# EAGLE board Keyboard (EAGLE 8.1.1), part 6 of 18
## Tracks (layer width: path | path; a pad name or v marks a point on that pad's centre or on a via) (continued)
S$5418 (continued)
  Bottom 0: 86.17,47.48 86.18,47.38
S$5419
  Bottom 0: 86.18,47.38 86.2,47.3
S$5420
  Bottom 0: 86.2,47.3 86.24,47.22
S$5421
  Bottom 0: 86.24,47.22 86.28,47.14
S$5422
  Bottom 0: 86.28,47.14 86.34,47.07
S$5423
  Bottom 0: 86.34,47.07 90.51,42.91
S$5424
  Bottom 0: 90.51,42.91 89.52,41.92
S$5425
  Bottom 0: 89.52,41.92 89.54,42.08
S$5426
  Bottom 0: 89.54,42.08 89.5,42.38
S$5427
  Bottom 0: 89.5,42.38 89.36,42.65
S$5428
  Bottom 0: 89.36,42.65 89.16,42.87
S$5429
  Bottom 0: 89.16,42.87 88.9,43.02
S$5430
  Bottom 0: 88.9,43.02 88.6,43.09
S$5431
  Bottom 0: 88.6,43.09 88.3,43.07
S$5432
  Bottom 0: 88.3,43.07 88.02,42.96
S$5433
  Bottom 0: 88.02,42.96 87.78,42.77
S$5434
  Bottom 0: 87.78,42.77 87.61,42.52
S$5435
  Bottom 0: 87.61,42.52 87.52,42.23
S$5436
  Bottom 0: 87.52,42.23 87.52,41.92
S$5437
  Bottom 0: 87.52,41.92 87.61,41.64
S$5438
  Bottom 0: 87.61,41.64 87.78,41.39
S$5439
  Bottom 0: 87.78,41.39 88.02,41.2
S$5440
  Bottom 0: 88.02,41.2 88.3,41.09
S$5441
  Bottom 0: 88.3,41.09 88.6,41.07
S$5442
  Bottom 0: 88.6,41.07 88.9,41.13
S$5443
  Bottom 0: 88.9,41.13 89.16,41.28
S$5444
  Bottom 0: 89.16,41.28 89.22,41.35
S$5445
  Bottom 0: 89.22,41.35 89.22,32.67
S$5446
  Bottom 0: 89.22,32.67 89.04,32.55
S$5447
  Bottom 0: 89.04,32.55 88.83,32.31
S$5448
  Bottom 0: 88.83,32.31 88.69,32.01
S$5449
  Bottom 0: 88.69,32.01 88.64,31.69
S$5450
  Bottom 0: 88.64,31.69 88.69,31.37
S$5451
  Bottom 0: 88.69,31.37 88.83,31.07
S$5452
  Bottom 0: 88.83,31.07 89.04,30.82
S$5453
  Bottom 0: 89.04,30.82 89.17,30.74
S$5454
  Bottom 0: 89.17,30.74 88.38,30.74
S$5455
  Bottom 0: 88.38,30.74 88.39,30.8
S$5456
  Bottom 0: 88.39,30.8 88.39,32.58
S$5457
  Bottom 0: 88.39,32.58 88.38,32.65
S$5458
  Bottom 0: 88.38,32.65 88.34,32.72
S$5459
  Bottom 0: 88.34,32.72 88.28,32.78
S$5460
  Bottom 0: 88.28,32.78 88.21,32.82
S$5461
  Bottom 0: 88.21,32.82 88.14,32.83
S$5462
  Bottom 0: 88.14,32.83 87.69,32.83
S$5463
  Bottom 0: 87.69,32.83 87.69,32.96
S$5464
  Bottom 0: 87.69,32.96 87.63,33.18
S$5465
  Bottom 0: 87.63,33.18 87.47,33.34
S$5466
  Bottom 0: 87.47,33.34 87.25,33.4
S$5467
  Bottom 0: 87.25,33.4 86.89,33.4
S$5468
  Bottom 0: 86.89,33.4 85.8,34.48
S$5469
  Bottom 0: 85.8,34.48 85.86,34.62
S$5470
  Bottom 0: 85.86,34.62 85.91,34.94
S$5471
  Bottom 0: 85.91,34.94 85.86,35.26
S$5472
  Bottom 0: 85.86,35.26 85.73,35.56
S$5473
  Bottom 0: 85.73,35.56 85.53,35.81
S$5474
  Bottom 0: 85.53,35.81 85.27,36
S$5475
  Bottom 0: 85.27,36 84.96,36.11
S$5476
  Bottom 0: 84.96,36.11 84.64,36.13
S$5477
  Bottom 0: 84.64,36.13 84.31,36.06
S$5478
  Bottom 0: 84.31,36.06 84.02,35.91
S$5479
  Bottom 0: 84.02,35.91 83.79,35.69
S$5480
  Bottom 0: 83.79,35.69 83.62,35.41
S$5481
  Bottom 0: 83.62,35.41 83.53,35.1
S$5482
  Bottom 0: 83.53,35.1 83.53,34.77
S$5483
  Bottom 0: 83.53,34.77 83.62,34.46
S$5484
  Bottom 0: 83.62,34.46 83.79,34.19
S$5485
  Bottom 0: 83.79,34.19 84.02,33.96
S$5486
  Bottom 0: 84.02,33.96 84.31,33.81
S$5487
  Bottom 0: 84.31,33.81 84.64,33.75
S$5488
  Bottom 0: 84.64,33.75 84.96,33.77
S$5489
  Bottom 0: 84.96,33.77 85.18,33.85
S$5490
  Bottom 0: 85.18,33.85 86.24,32.79
S$5491
  Bottom 0: 86.24,32.79 86.21,32.78
S$5492
  Bottom 0: 86.21,32.78 86.15,32.72
S$5493
  Bottom 0: 86.15,32.72 86.11,32.65
S$5494
  Bottom 0: 86.11,32.65 86.1,32.58
S$5495
  Bottom 0: 86.1,32.58 86.1,30.8
S$5496
  Bottom 0: 86.1,30.8 86.11,30.74
S$5497
  Bottom 0: 86.11,30.74 80,30.74
S$5498
  Bottom 0: 80,30.74 79.97,30.95
S$5499
  Bottom 0: 79.97,30.95 79.83,31.22
S$5500
  Bottom 0: 79.83,31.22 79.63,31.44
S$5501
  Bottom 0: 79.63,31.44 79.37,31.59
S$5502
  Bottom 0: 79.37,31.59 79.07,31.66
S$5503
  Bottom 0: 79.07,31.66 78.77,31.64
S$5504
  Bottom 0: 78.77,31.64 78.49,31.53
S$5505
  Bottom 0: 78.49,31.53 78.25,31.34
S$5506
  Bottom 0: 78.25,31.34 78.08,31.09
S$5507
  Bottom 0: 78.08,31.09 77.99,30.8
S$5508
  Bottom 0: 77.99,30.8 77.99,30.5
S$5509
  Bottom 0: 77.99,30.5 78.08,30.21
S$5510
  Bottom 0: 78.08,30.21 78.25,29.96
S$5511
  Bottom 0: 78.25,29.96 78.49,29.77
S$5512
  Bottom 0: 78.49,29.77 78.77,29.66
S$5513
  Bottom 0: 78.77,29.66 79.07,29.64
S$5514
  Bottom 0: 79.07,29.64 79.37,29.7
S$5515
  Bottom 0: 79.37,29.7 79.62,29.85
S$5516
  Bottom 0: 79.62,29.85 97.44,29.85
S$5517
  Bottom 0: 97.44,29.85 97.54,29.77
S$5518
  Bottom 0: 97.54,29.77 97.82,29.66
S$5519
  Bottom 0: 97.82,29.66 98.13,29.64
S$5520
  Bottom 0: 98.13,29.64 98.42,29.7
S$5521
  Bottom 0: 98.42,29.7 98.69,29.86
S$5522
  Bottom 0: 98.69,29.86 98.89,30.08
S$5523
  Bottom 0: 98.89,30.08 99.02,30.35
S$5524
  Bottom 0: 99.02,30.35 99.06,30.61
S$5525
  Bottom 0: 99.06,30.61 106.91,22.77
S$5526
  Bottom 0: 106.91,22.77 106.91,8.58
S$5527
  Bottom 0: 106.91,8.58 106.85,8.6
S$5528
  Bottom 0: 106.85,8.6 106.53,8.62
S$5529
  Bottom 0: 106.53,8.62 106.2,8.56
S$5530
  Bottom 0: 106.2,8.56 105.92,8.41
S$5531
  Bottom 0: 105.92,8.41 105.68,8.19
S$5532
  Bottom 0: 105.68,8.19 105.51,7.91
S$5533
  Bottom 0: 105.51,7.91 105.42,7.6
S$5534
  Bottom 0: 105.42,7.6 105.42,7.27
S$5535
  Bottom 0: 105.42,7.27 105.51,6.96
S$5536
  Bottom 0: 105.51,6.96 105.68,6.68
S$5537
  Bottom 0: 105.68,6.68 105.92,6.46
S$5538
  Bottom 0: 105.92,6.46 106.2,6.31
S$5539
  Bottom 0: 106.2,6.31 106.53,6.25
S$5540
  Bottom 0: 106.53,6.25 106.77,6.26
S$5541
  Bottom 0: 106.77,6.26 105.14,4.64
S$5542
  Bottom 0: 105.14,4.64 104.91,4.62
S$5543
  Bottom 0: 104.91,4.62 104.68,4.5
S$5544
  Bottom 0: 104.68,4.5 104.51,4.32
S$5545
  Bottom 0: 104.51,4.32 104.42,4.08
S$5546
  Bottom 0: 104.42,4.08 104.42,3.83
S$5547
  Bottom 0: 104.42,3.83 104.51,3.6
S$5548
  Bottom 0: 104.51,3.6 57.3,3.6
S$5549
  Bottom 0: 93.67,6.24 95.56,6.24
S$5550
  Bottom 0: 95.56,6.24 95.63,6.25
S$5551
  Bottom 0: 95.63,6.25 95.7,6.29
S$5552
  Bottom 0: 95.7,6.29 95.76,6.34
S$5553
  Bottom 0: 95.76,6.34 95.8,6.41
S$5554
  Bottom 0: 95.8,6.41 95.81,6.49
S$5555
  Bottom 0: 95.81,6.49 95.81,8.37
S$5556
  Bottom 0: 95.81,8.37 95.8,8.45
S$5557
  Bottom 0: 95.8,8.45 95.76,8.52
S$5558
  Bottom 0: 95.76,8.52 95.7,8.57
S$5559
  Bottom 0: 95.7,8.57 95.63,8.61
S$5560
  Bottom 0: 95.63,8.61 95.56,8.62
S$5561
  Bottom 0: 95.56,8.62 93.67,8.62
S$5562
  Bottom 0: 93.67,8.62 93.6,8.61
S$5563
  Bottom 0: 93.6,8.61 93.53,8.57
S$5564
  Bottom 0: 93.53,8.57 93.47,8.52
S$5565
  Bottom 0: 93.47,8.52 93.43,8.45
S$5566
  Bottom 0: 93.43,8.45 93.42,8.37
S$5567
  Bottom 0: 93.42,8.37 93.42,6.49
S$5568
  Bottom 0: 93.42,6.49 93.43,6.41
S$5569
  Bottom 0: 93.43,6.41 93.47,6.34
S$5570
  Bottom 0: 93.47,6.34 93.53,6.29
S$5571
  Bottom 0: 93.53,6.29 93.6,6.25
S$5572
  Bottom 0: 93.6,6.25 93.67,6.24
S$5573
  Bottom 0: 98.91,6.25 99.23,6.27
S$5574
  Bottom 0: 99.23,6.27 99.53,6.37
S$5575
  Bottom 0: 99.53,6.37 99.8,6.56
S$5576
  Bottom 0: 99.8,6.56 100.01,6.82
S$5577
  Bottom 0: 100.01,6.82 100.13,7.12
S$5578
  Bottom 0: 100.13,7.12 100.18,7.43
S$5579
  Bottom 0: 100.18,7.43 100.13,7.75
S$5580
  Bottom 0: 100.13,7.75 100.01,8.05
S$5581
  Bottom 0: 100.01,8.05 99.8,8.31
S$5582
  Bottom 0: 99.8,8.31 99.53,8.5
S$5583
  Bottom 0: 99.53,8.5 99.23,8.6
S$5584
  Bottom 0: 99.23,8.6 98.91,8.62
S$5585
  Bottom 0: 98.91,8.62 98.58,8.56
S$5586
  Bottom 0: 98.58,8.56 98.3,8.41
S$5587
  Bottom 0: 98.3,8.41 98.06,8.19
S$5588
  Bottom 0: 98.06,8.19 97.89,7.91
S$5589
  Bottom 0: 97.89,7.91 97.8,7.6
S$5590
  Bottom 0: 97.8,7.6 97.8,7.27
S$5591
  Bottom 0: 97.8,7.27 97.89,6.96
S$5592
  Bottom 0: 97.89,6.96 98.06,6.68
S$5593
  Bottom 0: 98.06,6.68 98.3,6.46
S$5594
  Bottom 0: 98.3,6.46 98.58,6.31
S$5595
  Bottom 0: 98.58,6.31 98.91,6.25
S$5596
  Bottom 0: 105.12,20.14 105.46,20.2
S$5597
  Bottom 0: 105.46,20.2 105.78,20.35
S$5598
  Bottom 0: 105.78,20.35 106.05,20.57
S$5599
  Bottom 0: 106.05,20.57 106.26,20.86
S$5600
  Bottom 0: 106.26,20.86 106.38,21.18
S$5601
  Bottom 0: 106.38,21.18 106.43,21.53
S$5602
  Bottom 0: 106.43,21.53 106.38,21.87
S$5603
  Bottom 0: 106.38,21.87 106.26,22.2
S$5604
  Bottom 0: 106.26,22.2 106.05,22.48
S$5605
  Bottom 0: 106.05,22.48 105.78,22.7
S$5606
  Bottom 0: 105.78,22.7 105.46,22.86
S$5607
  Bottom 0: 105.46,22.86 105.12,22.92
S$5608
  Bottom 0: 105.12,22.92 104.77,22.9
S$5609
  Bottom 0: 104.77,22.9 104.44,22.79
S$5610
  Bottom 0: 104.44,22.79 104.41,22.78
S$5611
  Bottom 0: 104.41,22.78 103.84,23.34
S$5612
  Bottom 0: 103.84,23.34 103.79,23.39
S$5613
  Bottom 0: 103.79,23.39 103.73,23.43
S$5614
  Bottom 0: 103.73,23.43 103.67,23.45
S$5615
  Bottom 0: 103.67,23.45 103.6,23.47
S$5616
  Bottom 0: 103.6,23.47 103.53,23.47
S$5617
  Bottom 0: 103.53,23.47 98.96,23.47
S$5618
  Bottom 0: 98.96,23.47 98.89,23.6
S$5619
  Bottom 0: 98.89,23.6 98.69,23.82
S$5620
  Bottom 0: 98.69,23.82 98.42,23.98
S$5621
  Bottom 0: 98.42,23.98 98.13,24.04
S$5622
  Bottom 0: 98.13,24.04 97.82,24.02
S$5623
  Bottom 0: 97.82,24.02 97.54,23.91
S$5624
  Bottom 0: 97.54,23.91 97.31,23.72
S$5625
  Bottom 0: 97.31,23.72 97.14,23.47
S$5626
  Bottom 0: 97.14,23.47 97.05,23.18
S$5627
  Bottom 0: 97.05,23.18 97.05,22.88
S$5628
  Bottom 0: 97.05,22.88 97.14,22.59
S$5629
  Bottom 0: 97.14,22.59 97.31,22.34
S$5630
  Bottom 0: 97.31,22.34 97.54,22.15
S$5631
  Bottom 0: 97.54,22.15 97.82,22.04
S$5632
  Bottom 0: 97.82,22.04 98.13,22.02
S$5633
  Bottom 0: 98.13,22.02 98.42,22.09
S$5634
  Bottom 0: 98.42,22.09 98.69,22.24
S$5635
  Bottom 0: 98.69,22.24 98.89,22.46
S$5636
  Bottom 0: 98.89,22.46 98.96,22.59
S$5637
  Bottom 0: 98.96,22.59 103.34,22.59
S$5638
  Bottom 0: 103.34,22.59 103.79,22.14
S$5639
  Bottom 0: 103.79,22.14 103.73,22.04
S$5640
  Bottom 0: 103.73,22.04 103.64,21.7
S$5641
  Bottom 0: 103.64,21.7 103.64,21.35
S$5642
  Bottom 0: 103.64,21.35 103.73,21.01
S$5643
  Bottom 0: 103.73,21.01 103.9,20.7
S$5644
  Bottom 0: 103.9,20.7 104.14,20.45
S$5645
  Bottom 0: 104.14,20.45 104.44,20.26
S$5646
  Bottom 0: 104.44,20.26 104.77,20.16
S$5647
  Bottom 0: 104.77,20.16 105.12,20.14
S$5648
  Bottom 0: 86.06,20.14 86.41,20.2
S$5649
  Bottom 0: 86.41,20.2 86.72,20.35
S$5650
  Bottom 0: 86.72,20.35 86.99,20.57
S$5651
  Bottom 0: 86.99,20.57 87.2,20.86
S$5652
  Bottom 0: 87.2,20.86 87.33,21.18
S$5653
  Bottom 0: 87.33,21.18 87.37,21.53
S$5654
  Bottom 0: 87.37,21.53 87.33,21.87
S$5655
  Bottom 0: 87.33,21.87 87.2,22.2
S$5656
  Bottom 0: 87.2,22.2 86.99,22.48
S$5657
  Bottom 0: 86.99,22.48 86.72,22.7
S$5658
  Bottom 0: 86.72,22.7 86.41,22.86
S$5659
  Bottom 0: 86.41,22.86 86.06,22.92
S$5660
  Bottom 0: 86.06,22.92 85.71,22.9
S$5661
  Bottom 0: 85.71,22.9 85.38,22.79
S$5662
  Bottom 0: 85.38,22.79 85.35,22.78
S$5663
  Bottom 0: 85.35,22.78 84.78,23.34
S$5664
  Bottom 0: 84.78,23.34 84.73,23.39
S$5665
  Bottom 0: 84.73,23.39 84.67,23.43
S$5666
  Bottom 0: 84.67,23.43 84.61,23.45
S$5667
  Bottom 0: 84.61,23.45 84.54,23.47
S$5668
  Bottom 0: 84.54,23.47 84.47,23.47
S$5669
  Bottom 0: 84.47,23.47 79.9,23.47
S$5670
  Bottom 0: 79.9,23.47 79.83,23.6
S$5671
  Bottom 0: 79.83,23.6 79.63,23.82
S$5672
  Bottom 0: 79.63,23.82 79.37,23.98
S$5673
  Bottom 0: 79.37,23.98 79.07,24.04
S$5674
  Bottom 0: 79.07,24.04 78.77,24.02
S$5675
  Bottom 0: 78.77,24.02 78.49,23.91
S$5676
  Bottom 0: 78.49,23.91 78.25,23.72
S$5677
  Bottom 0: 78.25,23.72 78.08,23.47
S$5678
  Bottom 0: 78.08,23.47 77.99,23.18
S$5679
  Bottom 0: 77.99,23.18 77.99,22.88
S$5680
  Bottom 0: 77.99,22.88 78.08,22.59
S$5681
  Bottom 0: 78.08,22.59 78.25,22.34
S$5682
  Bottom 0: 78.25,22.34 78.49,22.15
S$5683
  Bottom 0: 78.49,22.15 78.77,22.04
S$5684
  Bottom 0: 78.77,22.04 79.07,22.02
S$5685
  Bottom 0: 79.07,22.02 79.37,22.09
S$5686
  Bottom 0: 79.37,22.09 79.63,22.24
S$5687
  Bottom 0: 79.63,22.24 79.83,22.46
S$5688
  Bottom 0: 79.83,22.46 79.9,22.59
S$5689
  Bottom 0: 79.9,22.59 84.28,22.59
S$5690
  Bottom 0: 84.28,22.59 84.73,22.14
S$5691
  Bottom 0: 84.73,22.14 84.68,22.04
S$5692
  Bottom 0: 84.68,22.04 84.59,21.7
S$5693
  Bottom 0: 84.59,21.7 84.59,21.35
S$5694
  Bottom 0: 84.59,21.35 84.68,21.01
S$5695
  Bottom 0: 84.68,21.01 84.85,20.7
S$5696
  Bottom 0: 84.85,20.7 85.09,20.45
S$5697
  Bottom 0: 85.09,20.45 85.38,20.26
S$5698
  Bottom 0: 85.38,20.26 85.71,20.16
S$5699
  Bottom 0: 85.71,20.16 86.06,20.14
S$5700
  Bottom 0: 73.36,22.68 73.71,22.74
S$5701
  Bottom 0: 73.71,22.74 74.02,22.89
S$5702
  Bottom 0: 74.02,22.89 74.29,23.11
S$5703
  Bottom 0: 74.29,23.11 74.5,23.4
S$5704
  Bottom 0: 74.5,23.4 74.62,23.72
S$5705
  Bottom 0: 74.62,23.72 74.67,24.07
S$5706
  Bottom 0: 74.67,24.07 74.62,24.41
S$5707
  Bottom 0: 74.62,24.41 74.5,24.74
S$5708
  Bottom 0: 74.5,24.74 74.29,25.02
S$5709
  Bottom 0: 74.29,25.02 74.02,25.25
S$5710
  Bottom 0: 74.02,25.25 73.71,25.4
S$5711
  Bottom 0: 73.71,25.4 73.36,25.46
S$5712
  Bottom 0: 73.36,25.46 73.01,25.44
S$5713
  Bottom 0: 73.01,25.44 72.68,25.33
S$5714
  Bottom 0: 72.68,25.33 72.39,25.14
S$5715
  Bottom 0: 72.39,25.14 72.15,24.89
S$5716
  Bottom 0: 72.15,24.89 71.98,24.58
S$5717
  Bottom 0: 71.98,24.58 71.89,24.24
S$5718
  Bottom 0: 71.89,24.24 71.89,23.89
S$5719
  Bottom 0: 71.89,23.89 71.98,23.55
S$5720
  Bottom 0: 71.98,23.55 72.15,23.24
S$5721
  Bottom 0: 72.15,23.24 72.39,22.99
S$5722
  Bottom 0: 72.39,22.99 72.68,22.8
S$5723
  Bottom 0: 72.68,22.8 73.01,22.7
S$5724
  Bottom 0: 73.01,22.7 73.36,22.68
S$5725
  Bottom 0: 92.41,22.68 92.76,22.74
S$5726
  Bottom 0: 92.76,22.74 93.07,22.89
S$5727
  Bottom 0: 93.07,22.89 93.34,23.11
S$5728
  Bottom 0: 93.34,23.11 93.55,23.4
S$5729
  Bottom 0: 93.55,23.4 93.67,23.72
S$5730
  Bottom 0: 93.67,23.72 93.72,24.07
S$5731
  Bottom 0: 93.72,24.07 93.67,24.41
S$5732
  Bottom 0: 93.67,24.41 93.55,24.74
S$5733
  Bottom 0: 93.55,24.74 93.34,25.02
S$5734
  Bottom 0: 93.34,25.02 93.07,25.25
S$5735
  Bottom 0: 93.07,25.25 92.76,25.4
S$5736
  Bottom 0: 92.76,25.4 92.41,25.46
S$5737
  Bottom 0: 92.41,25.46 92.06,25.44
S$5738
  Bottom 0: 92.06,25.44 91.73,25.33
S$5739
  Bottom 0: 91.73,25.33 91.44,25.14
S$5740
  Bottom 0: 91.44,25.14 91.2,24.89
S$5741
  Bottom 0: 91.2,24.89 91.03,24.58
S$5742
  Bottom 0: 91.03,24.58 90.94,24.24
S$5743
  Bottom 0: 90.94,24.24 90.94,23.89
S$5744
  Bottom 0: 90.94,23.89 91.03,23.55
S$5745
  Bottom 0: 91.03,23.55 91.2,23.24
S$5746
  Bottom 0: 91.2,23.24 91.44,22.99
S$5747
  Bottom 0: 91.44,22.99 91.73,22.8
S$5748
  Bottom 0: 91.73,22.8 92.06,22.7
S$5749
  Bottom 0: 92.06,22.7 92.41,22.68
S$5750
  Bottom 0: 88.52,24.32 88.96,24.37
S$5751
  Bottom 0: 88.96,24.37 89.39,24.49
S$5752
  Bottom 0: 89.39,24.49 89.79,24.71
S$5753
  Bottom 0: 89.79,24.71 90.13,24.99
S$5754
  Bottom 0: 90.13,24.99 90.42,25.34
S$5755
  Bottom 0: 90.42,25.34 90.63,25.73
S$5756
  Bottom 0: 90.63,25.73 90.75,26.16
S$5757
  Bottom 0: 90.75,26.16 90.8,26.61
S$5758
  Bottom 0: 90.8,26.61 90.75,27.05
S$5759
  Bottom 0: 90.75,27.05 90.63,27.48
S$5760
  Bottom 0: 90.63,27.48 90.42,27.88
S$5761
  Bottom 0: 90.42,27.88 90.13,28.22
S$5762
  Bottom 0: 90.13,28.22 89.79,28.51
S$5763
  Bottom 0: 89.79,28.51 89.39,28.72
S$5764
  Bottom 0: 89.39,28.72 88.96,28.85
S$5765
  Bottom 0: 88.96,28.85 88.52,28.89
S$5766
  Bottom 0: 88.52,28.89 88.07,28.85
S$5767
  Bottom 0: 88.07,28.85 87.64,28.72
S$5768
  Bottom 0: 87.64,28.72 87.25,28.51
S$5769
  Bottom 0: 87.25,28.51 86.9,28.22
S$5770
  Bottom 0: 86.9,28.22 86.62,27.88
S$5771
  Bottom 0: 86.62,27.88 86.4,27.48
S$5772
  Bottom 0: 86.4,27.48 86.27,27.05
S$5773
  Bottom 0: 86.27,27.05 86.23,26.61
S$5774
  Bottom 0: 86.23,26.61 86.27,26.16
S$5775
  Bottom 0: 86.27,26.16 86.4,25.73
S$5776
  Bottom 0: 86.4,25.73 86.62,25.34
S$5777
  Bottom 0: 86.62,25.34 86.9,24.99
S$5778
  Bottom 0: 86.9,24.99 87.25,24.71
S$5779
  Bottom 0: 87.25,24.71 87.64,24.49
S$5780
  Bottom 0: 87.64,24.49 88.07,24.37
S$5781
  Bottom 0: 88.07,24.37 88.52,24.32
S$5782
  Bottom 0: 88.6,48.69 88.9,48.76
S$5783
  Bottom 0: 88.9,48.76 89.16,48.91
S$5784
  Bottom 0: 89.16,48.91 89.36,49.13
S$5785
  Bottom 0: 89.36,49.13 89.5,49.4
S$5786
  Bottom 0: 89.5,49.4 89.54,49.7
S$5787
  Bottom 0: 89.54,49.7 89.5,50
S$5788
  Bottom 0: 89.5,50 89.36,50.27
S$5789
  Bottom 0: 89.36,50.27 89.16,50.49
S$5790
  Bottom 0: 89.16,50.49 88.9,50.65
S$5791
  Bottom 0: 88.9,50.65 88.6,50.71
S$5792
  Bottom 0: 88.6,50.71 88.3,50.69
S$5793
  Bottom 0: 88.3,50.69 88.02,50.58
S$5794
  Bottom 0: 88.02,50.58 87.78,50.39
S$5795
  Bottom 0: 87.78,50.39 87.61,50.14
S$5796
  Bottom 0: 87.61,50.14 87.52,49.85
S$5797
  Bottom 0: 87.52,49.85 87.52,49.55
S$5798
  Bottom 0: 87.52,49.55 87.61,49.26
S$5799
  Bottom 0: 87.61,49.26 87.78,49.01
S$5800
  Bottom 0: 87.78,49.01 88.02,48.82
S$5801
  Bottom 0: 88.02,48.82 88.3,48.71
S$5802
  Bottom 0: 88.3,48.71 88.6,48.69
S$5803
  Bottom 0: 90.83,58.23 91.17,58.3
S$5804
  Bottom 0: 91.17,58.3 91.49,58.45
S$5805
  Bottom 0: 91.49,58.45 91.76,58.67
S$5806
  Bottom 0: 91.76,58.67 91.97,58.96
S$5807
  Bottom 0: 91.97,58.96 92.09,59.28
S$5808
  Bottom 0: 92.09,59.28 92.14,59.63
S$5809
  Bottom 0: 92.14,59.63 92.09,59.97
S$5810
  Bottom 0: 92.09,59.97 91.97,60.3
S$5811
  Bottom 0: 91.97,60.3 91.76,60.58
S$5812
  Bottom 0: 91.76,60.58 91.49,60.8
S$5813
  Bottom 0: 91.49,60.8 91.17,60.96
S$5814
  Bottom 0: 91.17,60.96 90.83,61.02
S$5815
  Bottom 0: 90.83,61.02 90.48,61
S$5816
  Bottom 0: 90.48,61 90.15,60.89
S$5817
  Bottom 0: 90.15,60.89 89.85,60.7
S$5818
  Bottom 0: 89.85,60.7 89.61,60.45
S$5819
  Bottom 0: 89.61,60.45 89.44,60.14
S$5820
  Bottom 0: 89.44,60.14 89.36,59.8
S$5821
  Bottom 0: 89.36,59.8 89.36,59.45
S$5822
  Bottom 0: 89.36,59.45 89.44,59.11
S$5823
  Bottom 0: 89.44,59.11 89.61,58.8
S$5824
  Bottom 0: 89.61,58.8 89.85,58.55
S$5825
  Bottom 0: 89.85,58.55 90.15,58.36
S$5826
  Bottom 0: 90.15,58.36 90.48,58.26
S$5827
  Bottom 0: 90.48,58.26 90.83,58.23
S$5828
  Bottom 0: 246.96,3.83 239.51,11.27
S$5829
  Bottom 0: 239.51,11.27 239.53,11.29
S$5830
  Bottom 0: 239.53,11.29 239.57,11.6
S$5831
  Bottom 0: 239.57,11.6 239.53,11.89
S$5832
  Bottom 0: 239.53,11.89 239.4,12.17
S$5833
  Bottom 0: 239.4,12.17 239.19,12.39
S$5834
  Bottom 0: 239.19,12.39 238.93,12.54
S$5835
  Bottom 0: 238.93,12.54 238.64,12.61
S$5836
  Bottom 0: 238.64,12.61 238.4,12.59
S$5837
  Bottom 0: 238.4,12.59 247.09,21.28
S$5838
  Bottom 0: 247.09,21.28 247.13,21.34
S$5839
  Bottom 0: 247.13,21.34 247.18,21.4
S$5840
  Bottom 0: 247.18,21.4 247.2,21.46
S$5841
  Bottom 0: 247.2,21.46 247.22,21.53
S$5842
  Bottom 0: 247.22,21.53 247.22,21.6
S$5843
  Bottom 0: 247.22,21.6 247.22,48.87
S$5844
  Bottom 0: 247.22,48.87 247.29,48.92
S$5845
  Bottom 0: 247.29,48.92 247.42,49.14
S$5846
  Bottom 0: 247.42,49.14 247.47,49.38
S$5847
  Bottom 0: 247.47,49.38 247.42,49.63
S$5848
  Bottom 0: 247.42,49.63 247.29,49.85
S$5849
  Bottom 0: 247.29,49.85 247.08,50
S$5850
  Bottom 0: 247.08,50 246.84,50.07
S$5851
  Bottom 0: 246.84,50.07 246.59,50.05
S$5852
  Bottom 0: 246.59,50.05 246.37,49.93
S$5853
  Bottom 0: 246.37,49.93 246.19,49.75
S$5854
  Bottom 0: 246.19,49.75 246.1,49.51
S$5855
  Bottom 0: 246.1,49.51 246.1,49.26
S$5856
  Bottom 0: 246.1,49.26 246.19,49.02
S$5857
  Bottom 0: 246.19,49.02 246.34,48.87
S$5858
  Bottom 0: 246.34,48.87 246.34,21.79
S$5859
  Bottom 0: 246.34,21.79 229.44,4.89
S$5860
  Bottom 0: 229.44,4.89 229.45,5.02
S$5861
  Bottom 0: 229.45,5.02 229.41,5.36
S$5862
  Bottom 0: 229.41,5.36 229.28,5.69
S$5863
  Bottom 0: 229.28,5.69 229.07,5.97
S$5864
  Bottom 0: 229.07,5.97 228.81,6.2
S$5865
  Bottom 0: 228.81,6.2 228.5,6.34
S$5866
  Bottom 0: 228.5,6.34 228.5,7.42
S$5867
  Bottom 0: 228.5,7.42 228.49,7.49
S$5868
  Bottom 0: 228.49,7.49 228.48,7.56
S$5869
  Bottom 0: 228.48,7.56 228.46,7.62
S$5870
  Bottom 0: 228.46,7.62 228.41,7.68
S$5871
  Bottom 0: 228.41,7.68 228.37,7.73
S$5872
  Bottom 0: 228.37,7.73 225.71,10.4
S$5873
  Bottom 0: 225.71,10.4 244.27,28.96
S$5874
  Bottom 0: 244.27,28.96 244.31,29.01
S$5875
  Bottom 0: 244.31,29.01 244.36,29.07
S$5876
  Bottom 0: 244.36,29.07 244.38,29.14
S$5877
  Bottom 0: 244.38,29.14 244.4,29.2
S$5878
  Bottom 0: 244.4,29.2 244.4,29.27
S$5879
  Bottom 0: 244.4,29.27 244.4,50.19
S$5880
  Bottom 0: 244.4,50.19 244.4,50.26
S$5881
  Bottom 0: 244.4,50.26 244.38,50.33
S$5882
  Bottom 0: 244.38,50.33 244.36,50.39
S$5883
  Bottom 0: 244.36,50.39 244.31,50.45
S$5884
  Bottom 0: 244.31,50.45 244.27,50.51
S$5885
  Bottom 0: 244.27,50.51 232.3,62.48
S$5886
  Bottom 0: 232.3,62.48 232.24,62.52
S$5887
  Bottom 0: 232.24,62.52 232.18,62.56
S$5888
  Bottom 0: 232.18,62.56 232.12,62.59
S$5889
  Bottom 0: 232.12,62.59 232.05,62.6
S$5890
  Bottom 0: 232.05,62.6 231.99,62.61
S$5891
  Bottom 0: 231.99,62.61 231.76,62.61
S$5892
  Bottom 0: 231.76,62.61 231.67,62.84
S$5893
  Bottom 0: 231.67,62.84 231.46,63.12
S$5894
  Bottom 0: 231.46,63.12 231.19,63.34
S$5895
  Bottom 0: 231.19,63.34 230.87,63.5
S$5896
  Bottom 0: 230.87,63.5 230.53,63.56
S$5897
  Bottom 0: 230.53,63.56 230.18,63.54
S$5898
  Bottom 0: 230.18,63.54 229.85,63.43
S$5899
  Bottom 0: 229.85,63.43 229.55,63.24
S$5900
  Bottom 0: 229.55,63.24 229.31,62.99
S$5901
  Bottom 0: 229.31,62.99 229.14,62.68
S$5902
  Bottom 0: 229.14,62.68 229.12,62.61
S$5903
  Bottom 0: 229.12,62.61 227.54,62.61
S$5904
  Bottom 0: 227.54,62.61 227.9,62.81
S$5905
  Bottom 0: 227.9,62.81 228.24,63.09
S$5906
  Bottom 0: 228.24,63.09 228.53,63.44
S$5907
  Bottom 0: 228.53,63.44 228.75,63.83
S$5908
  Bottom 0: 228.75,63.83 228.87,64.26
S$5909
  Bottom 0: 228.87,64.26 228.92,64.71
S$5910
  Bottom 0: 228.92,64.71 228.87,65.15
S$5911
  Bottom 0: 228.87,65.15 228.75,65.58
S$5912
  Bottom 0: 228.75,65.58 228.53,65.98
S$5913
  Bottom 0: 228.53,65.98 228.24,66.32
S$5914
  Bottom 0: 228.24,66.32 227.9,66.61
S$5915
  Bottom 0: 227.9,66.61 227.5,66.82
S$5916
  Bottom 0: 227.5,66.82 227.08,66.94
S$5917
  Bottom 0: 227.08,66.94 226.63,66.99
S$5918
  Bottom 0: 226.63,66.99 226.18,66.94
S$5919
  Bottom 0: 226.18,66.94 225.76,66.82
S$5920
  Bottom 0: 225.76,66.82 225.36,66.61
S$5921
  Bottom 0: 225.36,66.61 225.02,66.32
S$5922
  Bottom 0: 225.02,66.32 224.73,65.98
S$5923
  Bottom 0: 224.73,65.98 224.52,65.58
S$5924
  Bottom 0: 224.52,65.58 224.39,65.15
S$5925
  Bottom 0: 224.39,65.15 224.34,64.71
S$5926
  Bottom 0: 224.34,64.71 224.39,64.26
S$5927
  Bottom 0: 224.39,64.26 224.52,63.83
S$5928
  Bottom 0: 224.52,63.83 224.73,63.44
S$5929
  Bottom 0: 224.73,63.44 225.02,63.09
S$5930
  Bottom 0: 225.02,63.09 225.36,62.81
S$5931
  Bottom 0: 225.36,62.81 225.73,62.61
S$5932
  Bottom 0: 225.73,62.61 218.04,62.61
S$5933
  Bottom 0: 218.04,62.61 211.83,68.81
S$5934
  Bottom 0: 211.83,68.81 211.78,68.84
S$5935
  Bottom 0: 211.78,68.84 211.72,68.89
S$5936
  Bottom 0: 211.72,68.89 211.66,68.91
S$5937
  Bottom 0: 211.66,68.91 211.59,68.93
S$5938
  Bottom 0: 211.59,68.93 211.52,68.93
S$5939
  Bottom 0: 211.52,68.93 209.61,68.93
S$5940
  Bottom 0: 209.61,68.93 209.81,69.16
S$5941
  Bottom 0: 209.81,69.16 209.95,69.47
S$5942
  Bottom 0: 209.95,69.47 209.99,69.79
S$5943
  Bottom 0: 209.99,69.79 209.95,70.11
S$5944
  Bottom 0: 209.95,70.11 209.81,70.41
S$5945
  Bottom 0: 209.81,70.41 209.6,70.65
S$5946
  Bottom 0: 209.6,70.65 209.42,70.77
S$5947
  Bottom 0: 209.42,70.77 209.42,71.81
S$5948
  Bottom 0: 209.42,71.81 209.41,71.9
S$5949
  Bottom 0: 209.41,71.9 209.4,71.99
S$5950
  Bottom 0: 209.4,71.99 209.36,72.07
S$5951
  Bottom 0: 209.36,72.07 209.31,72.14
S$5952
  Bottom 0: 209.31,72.14 209.25,72.21
S$5953
  Bottom 0: 209.25,72.21 201.61,79.84
S$5954
  Bottom 0: 201.61,79.84 201.95,79.83
S$5955
  Bottom 0: 201.95,79.83 202.3,79.89
S$5956
  Bottom 0: 202.3,79.89 202.48,79.98
S$5957
  Bottom 0: 202.48,79.98 205.56,76.9
S$5958
  Bottom 0: 205.56,76.9 205.61,76.85
S$5959
  Bottom 0: 205.61,76.85 205.67,76.81
S$5960
  Bottom 0: 205.67,76.81 205.73,76.79
S$5961
  Bottom 0: 205.73,76.79 205.8,76.77
S$5962
  Bottom 0: 205.8,76.77 205.87,76.77
S$5963
  Bottom 0: 205.87,76.77 209.09,76.77
S$5964
  Bottom 0: 209.09,76.77 211.65,74.21
S$5965
  Bottom 0: 211.65,74.21 211.33,74.23
S$5966
  Bottom 0: 211.33,74.23 211.01,74.17
S$5967
  Bottom 0: 211.01,74.17 210.72,74.02
S$5968
  Bottom 0: 210.72,74.02 210.49,73.8
S$5969
  Bottom 0: 210.49,73.8 210.31,73.52
S$5970
  Bottom 0: 210.31,73.52 210.23,73.2
S$5971
  Bottom 0: 210.23,73.2 210.23,72.88
S$5972
  Bottom 0: 210.23,72.88 210.31,72.56
S$5973
  Bottom 0: 210.31,72.56 210.49,72.29
S$5974
  Bottom 0: 210.49,72.29 210.72,72.07
S$5975
  Bottom 0: 210.72,72.07 211.01,71.92
S$5976
  Bottom 0: 211.01,71.92 211.33,71.85
S$5977
  Bottom 0: 211.33,71.85 211.66,71.87
S$5978
  Bottom 0: 211.66,71.87 211.96,71.98
S$5979
  Bottom 0: 211.96,71.98 212.22,72.17
S$5980
  Bottom 0: 212.22,72.17 212.43,72.42
S$5981
  Bottom 0: 212.43,72.42 212.56,72.72
S$5982
  Bottom 0: 212.56,72.72 212.61,73.04
S$5983
  Bottom 0: 212.61,73.04 212.56,73.36
S$5984
  Bottom 0: 212.56,73.36 212.54,73.39
S$5985
  Bottom 0: 212.54,73.39 212.59,73.38
S$5986
  Bottom 0: 212.59,73.38 212.67,73.38
S$5987
  Bottom 0: 212.67,73.38 213.47,73.38
S$5988
  Bottom 0: 213.47,73.38 217.1,69.76
S$5989
  Bottom 0: 217.1,69.76 216.89,69.74
S$5990
  Bottom 0: 216.89,69.74 216.61,69.63
S$5991
  Bottom 0: 216.61,69.63 216.37,69.44
S$5992
  Bottom 0: 216.37,69.44 216.21,69.19
S$5993
  Bottom 0: 216.21,69.19 216.11,68.9
S$5994
  Bottom 0: 216.11,68.9 216.11,68.59
S$5995
  Bottom 0: 216.11,68.59 216.21,68.31
S$5996
  Bottom 0: 216.21,68.31 216.37,68.06
S$5997
  Bottom 0: 216.37,68.06 216.61,67.87
S$5998
  Bottom 0: 216.61,67.87 216.89,67.76
S$5999
  Bottom 0: 216.89,67.76 217.19,67.74
S$6000
  Bottom 0: 217.19,67.74 217.49,67.81
S$6001
  Bottom 0: 217.49,67.81 217.76,67.95
S$6002
  Bottom 0: 217.76,67.95 217.96,68.18
S$6003
  Bottom 0: 217.96,68.18 218.09,68.45
S$6004
  Bottom 0: 218.09,68.45 218.13,68.72
S$6005
  Bottom 0: 218.13,68.72 219.29,67.55
S$6006
  Bottom 0: 219.29,67.55 219.35,67.51
S$6007
  Bottom 0: 219.35,67.51 219.41,67.47
S$6008
  Bottom 0: 219.41,67.47 219.47,67.44
S$6009
  Bottom 0: 219.47,67.44 219.54,67.42
S$6010
  Bottom 0: 219.54,67.42 219.61,67.42
S$6011
  Bottom 0: 219.61,67.42 235.75,67.42
S$6012
  Bottom 0: 235.75,67.42 241.32,61.85
S$6013
  Bottom 0: 241.32,61.85 241.37,61.81
S$6014
  Bottom 0: 241.37,61.81 241.43,61.77
S$6015
  Bottom 0: 241.43,61.77 241.49,61.74
S$6016
  Bottom 0: 241.49,61.74 241.56,61.73
S$6017
  Bottom 0: 241.56,61.73 241.63,61.73
S$6018
  Bottom 0: 241.63,61.73 248.17,61.73
S$6019
  Bottom 0: 248.17,61.73 248.19,61.65
S$6020
  Bottom 0: 248.19,61.65 248.36,61.34
S$6021
  Bottom 0: 248.36,61.34 248.6,61.09
S$6022
  Bottom 0: 248.6,61.09 248.9,60.9
S$6023
  Bottom 0: 248.9,60.9 249.23,60.8
S$6024
  Bottom 0: 249.23,60.8 249.57,60.77
S$6025
  Bottom 0: 249.57,60.77 249.92,60.84
S$6026
  Bottom 0: 249.92,60.84 250.11,60.92
S$6027
  Bottom 0: 250.11,60.92 250.2,60.83
S$6028
  Bottom 0: 250.2,60.83 250.26,60.78
S$6029
  Bottom 0: 250.26,60.78 250.32,60.74
S$6030
  Bottom 0: 250.32,60.74 250.38,60.72
S$6031
  Bottom 0: 250.38,60.72 250.45,60.7
S$6032
  Bottom 0: 250.45,60.7 250.52,60.7
S$6033
  Bottom 0: 250.52,60.7 253.09,60.7
S$6034
  Bottom 0: 253.09,60.7 254.03,59.76
S$6035
  Bottom 0: 254.03,59.76 253.81,59.74
S$6036
  Bottom 0: 253.81,59.74 253.53,59.63
S$6037
  Bottom 0: 253.53,59.63 253.3,59.44
S$6038
  Bottom 0: 253.3,59.44 253.13,59.19
S$6039
  Bottom 0: 253.13,59.19 244.46,59.19
S$6040
  Bottom 0: 244.46,59.19 244.49,59.28
S$6041
  Bottom 0: 244.49,59.28 244.54,59.63
S$6042
  Bottom 0: 244.54,59.63 244.49,59.97
S$6043
  Bottom 0: 244.49,59.97 244.37,60.3
S$6044
  Bottom 0: 244.37,60.3 244.16,60.58
S$6045
  Bottom 0: 244.16,60.58 243.89,60.8
S$6046
  Bottom 0: 243.89,60.8 243.57,60.96
S$6047
  Bottom 0: 243.57,60.96 243.22,61.02
S$6048
  Bottom 0: 243.22,61.02 242.88,61
S$6049
  Bottom 0: 242.88,61 242.55,60.89
S$6050
  Bottom 0: 242.55,60.89 242.25,60.7
S$6051
  Bottom 0: 242.25,60.7 242.01,60.45
S$6052
  Bottom 0: 242.01,60.45 241.84,60.14
S$6053
  Bottom 0: 241.84,60.14 241.75,59.8
S$6054
  Bottom 0: 241.75,59.8 241.75,59.45
S$6055
  Bottom 0: 241.75,59.45 241.84,59.11
S$6056
  Bottom 0: 241.84,59.11 242.01,58.8
S$6057
  Bottom 0: 242.01,58.8 242.25,58.55
S$6058
  Bottom 0: 242.25,58.55 242.55,58.36
S$6059
  Bottom 0: 242.55,58.36 242.88,58.26
S$6060
  Bottom 0: 242.88,58.26 243.22,58.23
S$6061
  Bottom 0: 243.22,58.23 243.57,58.3
S$6062
  Bottom 0: 243.57,58.3 243.77,58.39
S$6063
  Bottom 0: 243.77,58.39 243.82,58.36
S$6064
  Bottom 0: 243.82,58.36 243.88,58.33
S$6065
  Bottom 0: 243.88,58.33 243.94,58.32
S$6066
  Bottom 0: 243.94,58.32 244.01,58.31
S$6067
  Bottom 0: 244.01,58.31 253.13,58.31
S$6068
  Bottom 0: 253.13,58.31 253.3,58.06
S$6069
  Bottom 0: 253.3,58.06 253.53,57.87
S$6070
  Bottom 0: 253.53,57.87 253.81,57.76
S$6071
  Bottom 0: 253.81,57.76 254.12,57.74
S$6072
  Bottom 0: 254.12,57.74 254.41,57.81
S$6073
  Bottom 0: 254.41,57.81 254.68,57.96
S$6074
  Bottom 0: 254.68,57.96 254.88,58.18
S$6075
  Bottom 0: 254.88,58.18 255.01,58.45
S$6076
  Bottom 0: 255.01,58.45 255.05,58.73
S$6077
  Bottom 0: 255.05,58.73 257.94,55.85
S$6078
  Bottom 0: 257.94,55.85 248.33,46.24
S$6079
  Bottom 0: 248.33,46.24 248.29,46.18
S$6080
  Bottom 0: 248.29,46.18 248.25,46.12
S$6081
  Bottom 0: 248.25,46.12 248.23,46.06
S$6082
  Bottom 0: 248.23,46.06 248.21,45.99
S$6083
  Bottom 0: 248.21,45.99 248.21,45.92
S$6084
  Bottom 0: 248.21,45.92 248.21,37.15
S$6085
  Bottom 0: 248.21,37.15 248.06,36.99
S$6086
  Bottom 0: 248.06,36.99 247.97,36.76
S$6087
  Bottom 0: 247.97,36.76 247.97,36.5
S$6088
  Bottom 0: 247.97,36.5 248.06,36.27
S$6089
  Bottom 0: 248.06,36.27 248.21,36.12
S$6090
  Bottom 0: 248.21,36.12 248.21,19.21
S$6091
  Bottom 0: 248.21,19.21 245.22,16.23
S$6092
  Bottom 0: 245.22,16.23 245.18,16.18
S$6093
  Bottom 0: 245.18,16.18 245.14,16.12
S$6094
  Bottom 0: 245.14,16.12 245.11,16.05
S$6095
  Bottom 0: 245.11,16.05 245.1,15.99
S$6096
  Bottom 0: 245.1,15.99 245.09,15.92
S$6097
  Bottom 0: 245.09,15.92 245.09,11.47
S$6098
  Bottom 0: 245.09,11.47 245.1,11.4
S$6099
  Bottom 0: 245.1,11.4 245.11,11.34
S$6100
  Bottom 0: 245.11,11.34 245.14,11.27
S$6101
  Bottom 0: 245.14,11.27 245.18,11.21
S$6102
  Bottom 0: 245.18,11.21 245.22,11.16
S$6103
  Bottom 0: 245.22,11.16 245.89,10.49
S$6104
  Bottom 0: 245.89,10.49 245.95,10.45
S$6105
  Bottom 0: 245.95,10.45 246.01,10.41
S$6106
  Bottom 0: 246.01,10.41 246.07,10.39
S$6107
  Bottom 0: 246.07,10.39 246.13,10.37
S$6108
  Bottom 0: 246.13,10.37 246.21,10.37
S$6109
  Bottom 0: 246.21,10.37 248.15,10.37
S$6110
  Bottom 0: 248.15,10.37 248.8,9.71
S$6111
  Bottom 0: 248.8,9.71 248.51,9.8
S$6112
  Bottom 0: 248.51,9.8 248.06,9.84
S$6113
  Bottom 0: 248.06,9.84 247.61,9.8
S$6114
  Bottom 0: 247.61,9.8 247.19,9.67
S$6115
  Bottom 0: 247.19,9.67 246.79,9.46
S$6116
  Bottom 0: 246.79,9.46 246.45,9.17
S$6117
  Bottom 0: 246.45,9.17 246.16,8.83
S$6118
  Bottom 0: 246.16,8.83 245.95,8.43
S$6119
  Bottom 0: 245.95,8.43 245.82,8
S$6120
  Bottom 0: 245.82,8 245.78,7.56
S$6121
  Bottom 0: 245.78,7.56 245.82,7.11
S$6122
  Bottom 0: 245.82,7.11 245.95,6.68
S$6123
  Bottom 0: 245.95,6.68 246.16,6.29
S$6124
  Bottom 0: 246.16,6.29 246.45,5.94
S$6125
  Bottom 0: 246.45,5.94 246.79,5.66
S$6126
  Bottom 0: 246.79,5.66 247.19,5.44
S$6127
  Bottom 0: 247.19,5.44 247.61,5.32
S$6128
  Bottom 0: 247.61,5.32 248.06,5.27
S$6129
  Bottom 0: 248.06,5.27 248.51,5.32
S$6130
  Bottom 0: 248.51,5.32 248.94,5.44
S$6131
  Bottom 0: 248.94,5.44 249.33,5.66
S$6132
  Bottom 0: 249.33,5.66 249.68,5.94
S$6133
  Bottom 0: 249.68,5.94 249.96,6.29
S$6134
  Bottom 0: 249.96,6.29 250.18,6.68
S$6135
  Bottom 0: 250.18,6.68 250.3,7.11
S$6136
  Bottom 0: 250.3,7.11 250.35,7.56
S$6137
  Bottom 0: 250.35,7.56 250.3,8
S$6138
  Bottom 0: 250.3,8 250.22,8.29
S$6139
  Bottom 0: 250.22,8.29 251.43,7.08
S$6140
  Bottom 0: 251.43,7.08 251.43,6.33
S$6141
  Bottom 0: 251.43,6.33 251.28,6.28
S$6142
  Bottom 0: 251.28,6.28 250.99,6.09
S$6143
  Bottom 0: 250.99,6.09 250.75,5.84
S$6144
  Bottom 0: 250.75,5.84 250.57,5.53
S$6145
  Bottom 0: 250.57,5.53 250.49,5.19
S$6146
  Bottom 0: 250.49,5.19 250.49,4.84
S$6147
  Bottom 0: 250.49,4.84 250.57,4.5
S$6148
  Bottom 0: 250.57,4.5 250.75,4.19
S$6149
  Bottom 0: 250.75,4.19 250.99,3.94
S$6150
  Bottom 0: 250.99,3.94 251.16,3.83
S$6151
  Bottom 0: 251.16,3.83 246.96,3.83
S$6152
  Bottom 0: 252.6,3.83 252.62,3.84
S$6153
  Bottom 0: 252.62,3.84 252.89,4.06
S$6154
  Bottom 0: 252.89,4.06 253.1,4.35
S$6155
  Bottom 0: 253.1,4.35 253.22,4.67
S$6156
  Bottom 0: 253.22,4.67 253.27,5.02
S$6157
  Bottom 0: 253.27,5.02 253.22,5.36
S$6158
  Bottom 0: 253.22,5.36 253.1,5.69
S$6159
  Bottom 0: 253.1,5.69 252.89,5.97
S$6160
  Bottom 0: 252.89,5.97 252.62,6.2
S$6161
  Bottom 0: 252.62,6.2 252.31,6.34
S$6162
  Bottom 0: 252.31,6.34 252.31,7.27
S$6163
  Bottom 0: 252.31,7.27 252.31,7.34
S$6164
  Bottom 0: 252.31,7.34 252.3,7.4
S$6165
  Bottom 0: 252.3,7.4 252.27,7.46
S$6166
  Bottom 0: 252.27,7.46 252.23,7.53
S$6167
  Bottom 0: 252.23,7.53 252.19,7.58
S$6168
  Bottom 0: 252.19,7.58 248.85,10.93
S$6169
  Bottom 0: 248.85,10.93 255.24,10.93
S$6170
  Bottom 0: 255.24,10.93 255.31,10.93
S$6171
  Bottom 0: 255.31,10.93 255.38,10.95
S$6172
  Bottom 0: 255.38,10.95 255.44,10.97
S$6173
  Bottom 0: 255.44,10.97 255.5,11.01
S$6174
  Bottom 0: 255.5,11.01 255.56,11.05
S$6175
  Bottom 0: 255.56,11.05 255.96,11.46
S$6176
  Bottom 0: 255.96,11.46 256.02,11.43
S$6177
  Bottom 0: 256.02,11.43 256.34,11.36
S$6178
  Bottom 0: 256.34,11.36 256.67,11.38
S$6179
  Bottom 0: 256.67,11.38 256.97,11.49
S$6180
  Bottom 0: 256.97,11.49 257.24,11.68
S$6181
  Bottom 0: 257.24,11.68 257.45,11.93
S$6182
  Bottom 0: 257.45,11.93 257.57,12.23
S$6183
  Bottom 0: 257.57,12.23 257.62,12.55
S$6184
  Bottom 0: 257.62,12.55 257.57,12.87
S$6185
  Bottom 0: 257.57,12.87 257.45,13.17
S$6186
  Bottom 0: 257.45,13.17 257.24,13.42
S$6187
  Bottom 0: 257.24,13.42 256.97,13.61
S$6188
  Bottom 0: 256.97,13.61 256.67,13.72
S$6189
  Bottom 0: 256.67,13.72 256.34,13.74
S$6190
  Bottom 0: 256.34,13.74 256.02,13.67
S$6191
  Bottom 0: 256.02,13.67 255.74,13.53
S$6192
  Bottom 0: 255.74,13.53 255.5,13.3
S$6193
  Bottom 0: 255.5,13.3 255.33,13.03
S$6194
  Bottom 0: 255.33,13.03 255.24,12.71
S$6195
  Bottom 0: 255.24,12.71 255.24,12.39
S$6196
  Bottom 0: 255.24,12.39 255.33,12.08
S$6197
  Bottom 0: 255.33,12.08 255.05,11.81
S$6198
  Bottom 0: 255.05,11.81 250.11,11.81
S$6199
  Bottom 0: 250.11,11.81 250.29,12.02
S$6200
  Bottom 0: 250.29,12.02 250.43,12.32
S$6201
  Bottom 0: 250.43,12.32 250.48,12.64
S$6202
  Bottom 0: 250.48,12.64 250.43,12.96
S$6203
  Bottom 0: 250.43,12.96 250.29,13.26
S$6204
  Bottom 0: 250.29,13.26 250.08,13.5
S$6205
  Bottom 0: 250.08,13.5 249.9,13.62
S$6206
  Bottom 0: 249.9,13.62 249.9,21.93
S$6207
  Bottom 0: 249.9,21.93 255.5,27.53
S$6208
  Bottom 0: 255.5,27.53 255.48,27.48
S$6209
  Bottom 0: 255.48,27.48 255.35,27.05
S$6210
  Bottom 0: 255.35,27.05 255.3,26.61
S$6211
  Bottom 0: 255.3,26.61 255.35,26.16
S$6212
  Bottom 0: 255.35,26.16 255.48,25.73
S$6213
  Bottom 0: 255.48,25.73 255.69,25.34
S$6214
  Bottom 0: 255.69,25.34 255.97,24.99
S$6215
  Bottom 0: 255.97,24.99 256.32,24.71
S$6216
  Bottom 0: 256.32,24.71 256.71,24.49
S$6217
  Bottom 0: 256.71,24.49 257.14,24.37
S$6218
  Bottom 0: 257.14,24.37 257.59,24.32
S$6219
  Bottom 0: 257.59,24.32 258.04,24.37
S$6220
  Bottom 0: 258.04,24.37 258.46,24.49
S$6221
  Bottom 0: 258.46,24.49 258.86,24.71
S$6222
  Bottom 0: 258.86,24.71 259.2,24.99
S$6223
  Bottom 0: 259.2,24.99 259.49,25.34
S$6224
  Bottom 0: 259.49,25.34 259.7,25.73
S$6225
  Bottom 0: 259.7,25.73 259.83,26.16
S$6226
  Bottom 0: 259.83,26.16 259.88,26.61
S$6227
  Bottom 0: 259.88,26.61 259.83,27.05
S$6228
  Bottom 0: 259.83,27.05 259.7,27.48
S$6229
  Bottom 0: 259.7,27.48 259.49,27.88
S$6230
  Bottom 0: 259.49,27.88 259.2,28.22
S$6231
  Bottom 0: 259.2,28.22 258.86,28.51
S$6232
  Bottom 0: 258.86,28.51 258.46,28.72
S$6233
  Bottom 0: 258.46,28.72 258.04,28.85
S$6234
  Bottom 0: 258.04,28.85 257.59,28.89
S$6235
  Bottom 0: 257.59,28.89 257.14,28.85
S$6236
  Bottom 0: 257.14,28.85 256.71,28.72
S$6237
  Bottom 0: 256.71,28.72 256.67,28.69
S$6238
  Bottom 0: 256.67,28.69 258.57,30.59
S$6239
  Bottom 0: 258.57,30.59 258.7,30.55
S$6240
  Bottom 0: 258.7,30.55 259.02,30.55
S$6241
  Bottom 0: 259.02,30.55 259.33,30.64
S$6242
  Bottom 0: 259.33,30.64 259.61,30.82
S$6243
  Bottom 0: 259.61,30.82 259.82,31.07
S$6244
  Bottom 0: 259.82,31.07 259.96,31.37
S$6245
  Bottom 0: 259.96,31.37 260,31.69
S$6246
  Bottom 0: 260,31.69 259.96,32.01
S$6247
  Bottom 0: 259.96,32.01 259.82,32.31
S$6248
  Bottom 0: 259.82,32.31 259.61,32.55
S$6249
  Bottom 0: 259.61,32.55 259.33,32.73
S$6250
  Bottom 0: 259.33,32.73 259.02,32.82
S$6251
  Bottom 0: 259.02,32.82 258.7,32.82
S$6252
  Bottom 0: 258.7,32.82 258.56,32.78
S$6253
  Bottom 0: 258.56,32.78 258.52,32.82
S$6254
  Bottom 0: 258.52,32.82 258.52,40.04
S$6255
  Bottom 0: 258.52,40.04 258.68,39.75
S$6256
  Bottom 0: 258.68,39.75 258.92,39.5
S$6257
  Bottom 0: 258.92,39.5 259.21,39.31
S$6258
  Bottom 0: 259.21,39.31 259.55,39.2
S$6259
  Bottom 0: 259.55,39.2 259.89,39.19
S$6260
  Bottom 0: 259.89,39.19 260.24,39.25
S$6261
  Bottom 0: 260.24,39.25 260.56,39.4
S$6262
  Bottom 0: 260.56,39.4 260.82,39.62
S$6263
  Bottom 0: 260.82,39.62 261.03,39.91
S$6264
  Bottom 0: 261.03,39.91 261.16,40.23
S$6265
  Bottom 0: 261.16,40.23 261.2,40.58
S$6266
  Bottom 0: 261.2,40.58 261.16,40.92
S$6267
  Bottom 0: 261.16,40.92 261.03,41.25
S$6268
  Bottom 0: 261.03,41.25 260.82,41.53
S$6269
  Bottom 0: 260.82,41.53 260.56,41.76
S$6270
  Bottom 0: 260.56,41.76 260.24,41.91
S$6271
  Bottom 0: 260.24,41.91 259.89,41.97
S$6272
  Bottom 0: 259.89,41.97 259.55,41.95
S$6273
  Bottom 0: 259.55,41.95 259.21,41.84
S$6274
  Bottom 0: 259.21,41.84 258.92,41.65
S$6275
  Bottom 0: 258.92,41.65 258.68,41.4
S$6276
  Bottom 0: 258.68,41.4 258.52,41.11
S$6277
  Bottom 0: 258.52,41.11 258.52,44.83
S$6278
  Bottom 0: 258.52,44.83 260.26,46.58
S$6279
  Bottom 0: 260.26,46.58 260.24,46.53
S$6280
  Bottom 0: 260.24,46.53 260.11,46.1
S$6281
  Bottom 0: 260.11,46.1 260.06,45.66
S$6282
  Bottom 0: 260.06,45.66 260.11,45.21
S$6283
  Bottom 0: 260.11,45.21 260.24,44.78
S$6284
  Bottom 0: 260.24,44.78 260.45,44.39
S$6285
  Bottom 0: 260.45,44.39 260.73,44.04
S$6286
  Bottom 0: 260.73,44.04 261.08,43.76
S$6287
  Bottom 0: 261.08,43.76 261.48,43.54
S$6288
  Bottom 0: 261.48,43.54 261.9,43.42
S$6289
  Bottom 0: 261.9,43.42 262.35,43.37
S$6290
  Bottom 0: 262.35,43.37 262.8,43.42
S$6291
  Bottom 0: 262.8,43.42 263.22,43.54
S$6292
  Bottom 0: 263.22,43.54 263.62,43.76
S$6293
  Bottom 0: 263.62,43.76 263.96,44.04
S$6294
  Bottom 0: 263.96,44.04 264.25,44.39
S$6295
  Bottom 0: 264.25,44.39 264.46,44.78
S$6296
  Bottom 0: 264.46,44.78 264.59,45.21
S$6297
  Bottom 0: 264.59,45.21 264.63,45.66
S$6298
  Bottom 0: 264.63,45.66 264.59,46.1
S$6299
  Bottom 0: 264.59,46.1 264.46,46.53
S$6300
  Bottom 0: 264.46,46.53 264.25,46.93
S$6301
  Bottom 0: 264.25,46.93 263.96,47.27
S$6302
  Bottom 0: 263.96,47.27 263.62,47.56
S$6303
  Bottom 0: 263.62,47.56 263.22,47.77
S$6304
  Bottom 0: 263.22,47.77 262.8,47.89
S$6305
  Bottom 0: 262.8,47.89 262.35,47.94
S$6306
  Bottom 0: 262.35,47.94 261.9,47.89
S$6307
  Bottom 0: 261.9,47.89 261.48,47.77
S$6308
  Bottom 0: 261.48,47.77 261.43,47.74
S$6309
  Bottom 0: 261.43,47.74 263.33,49.64
S$6310
  Bottom 0: 263.33,49.64 263.46,49.6
S$6311
  Bottom 0: 263.46,49.6 263.78,49.6
S$6312
  Bottom 0: 263.78,49.6 264.09,49.7
S$6313
  Bottom 0: 264.09,49.7 264.37,49.87
S$6314
  Bottom 0: 264.37,49.87 264.58,50.11
S$6315
  Bottom 0: 264.58,50.11 264.72,50.42
S$6316
  Bottom 0: 264.72,50.42 264.76,50.74
S$6317
  Bottom 0: 264.76,50.74 264.72,51.06
S$6318
  Bottom 0: 264.72,51.06 264.58,51.36
S$6319
  Bottom 0: 264.58,51.36 264.37,51.6
S$6320
  Bottom 0: 264.37,51.6 264.09,51.78
S$6321
  Bottom 0: 264.09,51.78 263.78,51.87
S$6322
  Bottom 0: 263.78,51.87 263.46,51.87
S$6323
  Bottom 0: 263.46,51.87 263.15,51.78
S$6324
  Bottom 0: 263.15,51.78 262.87,51.6
S$6325
  Bottom 0: 262.87,51.6 262.66,51.36
S$6326
  Bottom 0: 262.66,51.36 262.52,51.06
S$6327
  Bottom 0: 262.52,51.06 262.47,50.74
S$6328
  Bottom 0: 262.47,50.74 262.52,50.43
S$6329
  Bottom 0: 262.52,50.43 262.22,50.14
S$6330
  Bottom 0: 262.22,50.14 262.22,51.63
S$6331
  Bottom 0: 262.22,51.63 262.21,51.7
S$6332
  Bottom 0: 262.21,51.7 262.17,51.77
S$6333
  Bottom 0: 262.17,51.77 262.12,51.83
S$6334
  Bottom 0: 262.12,51.83 262.04,51.87
S$6335
  Bottom 0: 262.04,51.87 261.96,51.88
S$6336
  Bottom 0: 261.96,51.88 261.52,51.88
S$6337
  Bottom 0: 261.52,51.88 261.52,52.01
S$6338
  Bottom 0: 261.52,52.01 261.46,52.23
S$6339
  Bottom 0: 261.46,52.23 261.3,52.39
S$6340
  Bottom 0: 261.3,52.39 261.08,52.45
S$6341
  Bottom 0: 261.08,52.45 260.74,52.45
S$6342
  Bottom 0: 260.74,52.45 259.66,53.54
S$6343
  Bottom 0: 259.66,53.54 259.72,53.67
S$6344
  Bottom 0: 259.72,53.67 259.76,53.99
S$6345
  Bottom 0: 259.76,53.99 259.76,54.02
S$6346
  Bottom 0: 259.76,54.02 261.56,52.23
S$6347
  Bottom 0: 261.56,52.23 261.61,52.18
S$6348
  Bottom 0: 261.61,52.18 261.67,52.14
S$6349
  Bottom 0: 261.67,52.14 261.73,52.12
S$6350
  Bottom 0: 261.73,52.12 261.8,52.1
S$6351
  Bottom 0: 261.8,52.1 261.87,52.1
S$6352
  Bottom 0: 261.87,52.1 279.47,52.1
S$6353
  Bottom 0: 279.47,52.1 279.53,52.1
S$6354
  Bottom 0: 279.53,52.1 261.35,33.93
S$6355
  Bottom 0: 261.35,33.93 261.31,33.87
S$6356
  Bottom 0: 261.31,33.87 261.27,33.81
S$6357
  Bottom 0: 261.27,33.81 261.25,33.75
S$6358
  Bottom 0: 261.25,33.75 261.23,33.68
S$6359
  Bottom 0: 261.23,33.68 261.23,33.61
S$6360
  Bottom 0: 261.23,33.61 261.23,28.22
S$6361
  Bottom 0: 261.23,28.22 261.18,28.26
S$6362
  Bottom 0: 261.18,28.26 260.93,28.32
S$6363
  Bottom 0: 260.93,28.32 260.68,28.3
S$6364
  Bottom 0: 260.68,28.3 260.46,28.19
S$6365
  Bottom 0: 260.46,28.19 260.29,28
S$6366
  Bottom 0: 260.29,28 260.19,27.77
S$6367
  Bottom 0: 260.19,27.77 260.19,27.52
S$6368
  Bottom 0: 260.19,27.52 260.29,27.28
S$6369
  Bottom 0: 260.29,27.28 260.42,27.14
S$6370
  Bottom 0: 260.42,27.14 260.42,26.1
S$6371
  Bottom 0: 260.42,26.1 259.49,25.17
S$6372
  Bottom 0: 259.49,25.17 259.45,25.11
S$6373
  Bottom 0: 259.45,25.11 259.41,25.05
S$6374
  Bottom 0: 259.41,25.05 259.39,24.99
S$6375
  Bottom 0: 259.39,24.99 259.37,24.93
S$6376
  Bottom 0: 259.37,24.93 259.37,24.85
S$6377
  Bottom 0: 259.37,24.85 259.37,23.41
S$6378
  Bottom 0: 259.37,23.41 259.37,23.34
S$6379
  Bottom 0: 259.37,23.34 259.39,23.28
S$6380
  Bottom 0: 259.39,23.28 259.41,23.21
S$6381
  Bottom 0: 259.41,23.21 259.45,23.16
S$6382
  Bottom 0: 259.45,23.16 259.49,23.1
S$6383
  Bottom 0: 259.49,23.1 259.58,23.02
S$6384
  Bottom 0: 259.58,23.02 259.58,14.14
S$6385
  Bottom 0: 259.58,14.14 259.44,14.29
S$6386
  Bottom 0: 259.44,14.29 259.25,14.4
S$6387
  Bottom 0: 259.25,14.4 259.25,17.77
S$6388
  Bottom 0: 259.25,17.77 259.24,17.84
S$6389
  Bottom 0: 259.24,17.84 259.23,17.91
S$6390
  Bottom 0: 259.23,17.91 259.2,17.97
S$6391
  Bottom 0: 259.2,17.97 259.16,18.03
S$6392
  Bottom 0: 259.16,18.03 259.12,18.09
S$6393
  Bottom 0: 259.12,18.09 256.29,20.91
S$6394
  Bottom 0: 256.29,20.91 256.4,21.18
S$6395
  Bottom 0: 256.4,21.18 256.45,21.53
S$6396
  Bottom 0: 256.45,21.53 256.4,21.87
S$6397
  Bottom 0: 256.4,21.87 256.27,22.2
S$6398
  Bottom 0: 256.27,22.2 256.06,22.48
S$6399
  Bottom 0: 256.06,22.48 255.8,22.7
S$6400
  Bottom 0: 255.8,22.7 255.48,22.86
S$6401
  Bottom 0: 255.48,22.86 255.13,22.92
S$6402
  Bottom 0: 255.13,22.92 254.78,22.9
S$6403
  Bottom 0: 254.78,22.9 254.46,22.79
S$6404
  Bottom 0: 254.46,22.79 254.16,22.6
S$6405
  Bottom 0: 254.16,22.6 253.92,22.35
S$6406
  Bottom 0: 253.92,22.35 253.75,22.04
S$6407
  Bottom 0: 253.75,22.04 253.66,21.7
S$6408
  Bottom 0: 253.66,21.7 253.66,21.35
S$6409
  Bottom 0: 253.66,21.35 253.75,21.01
S$6410
  Bottom 0: 253.75,21.01 253.92,20.7
S$6411
  Bottom 0: 253.92,20.7 254.16,20.45
S$6412
  Bottom 0: 254.16,20.45 254.46,20.26
S$6413
  Bottom 0: 254.46,20.26 254.78,20.16
S$6414
  Bottom 0: 254.78,20.16 255.13,20.14
S$6415
  Bottom 0: 255.13,20.14 255.48,20.2
S$6416
  Bottom 0: 255.48,20.2 255.66,20.28
S$6417
  Bottom 0: 255.66,20.28 258.36,17.58
S$6418
  Bottom 0: 258.36,17.58 258.36,14.4
S$6419
  Bottom 0: 258.36,14.4 258.3,14.38
S$6420
  Bottom 0: 258.3,14.38 258.06,14.19
S$6421
  Bottom 0: 258.06,14.19 257.89,13.94
S$6422
  Bottom 0: 257.89,13.94 257.8,13.65
S$6423
  Bottom 0: 257.8,13.65 257.8,13.35
S$6424
  Bottom 0: 257.8,13.35 257.89,13.06
S$6425
  Bottom 0: 257.89,13.06 258.06,12.81
S$6426
  Bottom 0: 258.06,12.81 258.3,12.62
S$6427
  Bottom 0: 258.3,12.62 258.57,12.51
S$6428
  Bottom 0: 258.57,12.51 258.88,12.49
S$6429
  Bottom 0: 258.88,12.49 259.17,12.55
S$6430
  Bottom 0: 259.17,12.55 259.44,12.71
S$6431
  Bottom 0: 259.44,12.71 259.58,12.86
S$6432
  Bottom 0: 259.58,12.86 259.58,7.29
S$6433
  Bottom 0: 259.58,7.29 259.13,6.83
S$6434
  Bottom 0: 259.13,6.83 258.88,6.89
S$6435
  Bottom 0: 258.88,6.89 258.57,6.87
S$6436
  Bottom 0: 258.57,6.87 258.3,6.76
S$6437
  Bottom 0: 258.3,6.76 258.06,6.57
S$6438
  Bottom 0: 258.06,6.57 257.89,6.32
S$6439
  Bottom 0: 257.89,6.32 257.8,6.03
S$6440
  Bottom 0: 257.8,6.03 257.8,5.73
S$6441
  Bottom 0: 257.8,5.73 257.89,5.44
S$6442
  Bottom 0: 257.89,5.44 258.06,5.19
S$6443
  Bottom 0: 258.06,5.19 258.3,5
S$6444
  Bottom 0: 258.3,5 258.57,4.89
S$6445
  Bottom 0: 258.57,4.89 258.88,4.87
S$6446
  Bottom 0: 258.88,4.87 259.17,4.93
S$6447
  Bottom 0: 259.17,4.93 259.44,5.09
S$6448
  Bottom 0: 259.44,5.09 259.64,5.31
S$6449
  Bottom 0: 259.64,5.31 259.77,5.58
S$6450
  Bottom 0: 259.77,5.58 259.82,5.88
S$6451
  Bottom 0: 259.82,5.88 259.77,6.18
S$6452
  Bottom 0: 259.77,6.18 259.76,6.21
S$6453
  Bottom 0: 259.76,6.21 260.34,6.79
S$6454
  Bottom 0: 260.34,6.79 260.38,6.84
S$6455
  Bottom 0: 260.38,6.84 260.42,6.91
S$6456
  Bottom 0: 260.42,6.91 260.44,6.97
S$6457
  Bottom 0: 260.44,6.97 260.46,7.03
S$6458
  Bottom 0: 260.46,7.03 260.46,7.1
S$6459
  Bottom 0: 260.46,7.1 260.46,23.04
S$6460
  Bottom 0: 260.46,23.04 260.51,22.99
S$6461
  Bottom 0: 260.51,22.99 260.81,22.8
S$6462
  Bottom 0: 260.81,22.8 261.13,22.7
S$6463
  Bottom 0: 261.13,22.7 261.49,22.68
S$6464
  Bottom 0: 261.49,22.68 261.83,22.74
S$6465
  Bottom 0: 261.83,22.74 262.01,22.82
S$6466
  Bottom 0: 262.01,22.82 270.39,14.45
S$6467
  Bottom 0: 270.39,14.45 270.39,12.11
S$6468
  Bottom 0: 270.39,12.11 270.36,12.17
S$6469
  Bottom 0: 270.36,12.17 270.15,12.39
S$6470
  Bottom 0: 270.15,12.39 269.89,12.54
S$6471
  Bottom 0: 269.89,12.54 269.6,12.61
S$6472
  Bottom 0: 269.6,12.61 269.29,12.59
S$6473
  Bottom 0: 269.29,12.59 269.01,12.47
S$6474
  Bottom 0: 269.01,12.47 268.77,12.29
S$6475
  Bottom 0: 268.77,12.29 268.61,12.04
S$6476
  Bottom 0: 268.61,12.04 268.52,11.75
S$6477
  Bottom 0: 268.52,11.75 268.52,11.44
S$6478
  Bottom 0: 268.52,11.44 268.57,11.27
S$6479
  Bottom 0: 268.57,11.27 261.12,3.83
S$6480
  Bottom 0: 261.12,3.83 256.86,3.83
S$6481
  Bottom 0: 256.86,3.83 256.97,3.87
S$6482
  Bottom 0: 256.97,3.87 257.24,4.06
S$6483
  Bottom 0: 257.24,4.06 257.45,4.31
S$6484
  Bottom 0: 257.45,4.31 257.57,4.61
S$6485
  Bottom 0: 257.57,4.61 257.62,4.93
S$6486
  Bottom 0: 257.62,4.93 257.57,5.25
S$6487
  Bottom 0: 257.57,5.25 257.45,5.55
S$6488
  Bottom 0: 257.45,5.55 257.24,5.8
S$6489
  Bottom 0: 257.24,5.8 256.97,5.99
S$6490
  Bottom 0: 256.97,5.99 256.67,6.1
S$6491
  Bottom 0: 256.67,6.1 256.34,6.12
S$6492
  Bottom 0: 256.34,6.12 256.02,6.05
S$6493
  Bottom 0: 256.02,6.05 255.74,5.91
S$6494
  Bottom 0: 255.74,5.91 255.5,5.68
S$6495
  Bottom 0: 255.5,5.68 255.33,5.41
S$6496
  Bottom 0: 255.33,5.41 255.24,5.09
S$6497
  Bottom 0: 255.24,5.09 255.24,4.77
S$6498
  Bottom 0: 255.24,4.77 255.33,4.45
S$6499
  Bottom 0: 255.33,4.45 255.5,4.18
S$6500
  Bottom 0: 255.5,4.18 255.74,3.96
S$6501
  Bottom 0: 255.74,3.96 255.98,3.83
S$6502
  Bottom 0: 255.98,3.83 252.6,3.83
S$6503
  Bottom 0: 266.25,41.73 266.59,41.79
S$6504
  Bottom 0: 266.59,41.79 266.91,41.94
S$6505
  Bottom 0: 266.91,41.94 267.17,42.16
S$6506
  Bottom 0: 267.17,42.16 267.38,42.45
S$6507
  Bottom 0: 267.38,42.45 267.51,42.77
S$6508
  Bottom 0: 267.51,42.77 267.55,43.12
S$6509
  Bottom 0: 267.55,43.12 267.51,43.46
S$6510
  Bottom 0: 267.51,43.46 267.4,43.73
S$6511
  Bottom 0: 267.4,43.73 273.29,49.61
S$6512
  Bottom 0: 273.29,49.61 273.39,49.6
S$6513
  Bottom 0: 273.39,49.6 273.63,49.67
S$6514
  Bottom 0: 273.63,49.67 273.83,49.82
S$6515
  Bottom 0: 273.83,49.82 273.96,50.03
S$6516
  Bottom 0: 273.96,50.03 274.01,50.28
S$6517
  Bottom 0: 274.01,50.28 273.96,50.53
S$6518
  Bottom 0: 273.96,50.53 273.83,50.75
S$6519
  Bottom 0: 273.83,50.75 273.63,50.9
S$6520
  Bottom 0: 273.63,50.9 273.39,50.97
S$6521
  Bottom 0: 273.39,50.97 273.14,50.94
S$6522
  Bottom 0: 273.14,50.94 272.92,50.83
S$6523
  Bottom 0: 272.92,50.83 272.74,50.65
S$6524
  Bottom 0: 272.74,50.65 272.65,50.41
S$6525
  Bottom 0: 272.65,50.41 272.65,50.24
S$6526
  Bottom 0: 272.65,50.24 266.77,44.36
S$6527
  Bottom 0: 266.77,44.36 266.59,44.45
S$6528
  Bottom 0: 266.59,44.45 266.25,44.51
S$6529
  Bottom 0: 266.25,44.51 265.89,44.49
S$6530
  Bottom 0: 265.89,44.49 265.56,44.38
S$6531
  Bottom 0: 265.56,44.38 265.27,44.19
S$6532
  Bottom 0: 265.27,44.19 265.03,43.94
S$6533
  Bottom 0: 265.03,43.94 264.86,43.63
S$6534
  Bottom 0: 264.86,43.63 264.77,43.29
S$6535
  Bottom 0: 264.77,43.29 264.77,42.94
S$6536
  Bottom 0: 264.77,42.94 264.86,42.6
S$6537
  Bottom 0: 264.86,42.6 265.03,42.29
S$6538
  Bottom 0: 265.03,42.29 265.27,42.04
S$6539
  Bottom 0: 265.27,42.04 265.56,41.85
S$6540
  Bottom 0: 265.56,41.85 265.89,41.74
S$6541
  Bottom 0: 265.89,41.74 266.25,41.73
S$6542
  Bottom 0: 105.77,4
S$6543
  Bottom 0: 105.77,4 111.7,9.93
S$6544
  Bottom 0: 111.7,9.93 111.74,9.98
S$6545
  Bottom 0: 111.74,9.98 111.78,10.05
S$6546
  Bottom 0: 111.78,10.05 111.8,10.11
S$6547
  Bottom 0: 111.8,10.11 111.82,10.17
S$6548
  Bottom 0: 111.82,10.17 111.82,10.24
S$6549
  Bottom 0: 111.82,10.24 111.82,22.74
S$6550
  Bottom 0: 111.82,22.74 112.13,22.89
S$6551
  Bottom 0: 112.13,22.89 112.4,23.11
S$6552
  Bottom 0: 112.4,23.11 112.61,23.4
S$6553
  Bottom 0: 112.61,23.4 112.73,23.72
S$6554
  Bottom 0: 112.73,23.72 112.78,24.07
S$6555
  Bottom 0: 112.78,24.07 112.73,24.41
S$6556
  Bottom 0: 112.73,24.41 112.61,24.74
S$6557
  Bottom 0: 112.61,24.74 112.4,25.02
S$6558
  Bottom 0: 112.4,25.02 112.13,25.25
S$6559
